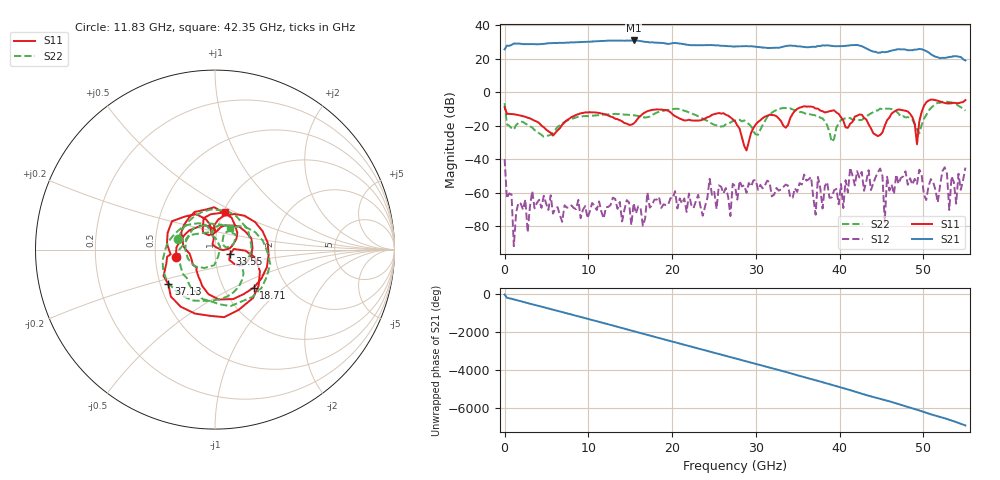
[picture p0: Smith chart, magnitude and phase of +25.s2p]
!Agilent Technologies,E8361C,US49010292,A.09.42.06
!Agilent E8361C: A.09.42.06
!Date: Thursday, December 21, 2023 21:15:18
!Correction: S11(Full 2 Port(1,2))
!S21(Full 2 Port(1,2))
!S12(Full 2 Port(1,2))
!S22(Full 2 Port(1,2))
!S2P File: Measurements: S11, S21, S12, S22:
# Hz S  dB  R 50
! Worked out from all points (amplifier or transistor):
!   201 points, 10 MHz to 55 GHz, reference 50 ohm
!   highest |S21| = 30.9 dB at 15.41 GHz (marker M1)
!   |S21| within 3 dB of that: 674.4 MHz to 25.59 GHz (24.92 GHz wide, 190 % of centre)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
!   unconditionally stable (mu >= 1): start of sweep to end of sweep
!   at 9.083 GHz: K = 84.46, MAG = 30.4 dB, |S12| = -75.3 dB
!   at 27.5 GHz: K = 13.18, MAG = 27.4 dB, |S12| = -56.0 dB
!   at 55 GHz: K = 6.36, MAG = 21.0 dB, |S12| = -45.1 dB
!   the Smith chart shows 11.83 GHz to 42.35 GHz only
!   S11 on the Smith chart (normalised r, x): 11.83 GHz: 0.64, -0.06; 18.71 GHz: 1.38, -0.64; 33.55 GHz: 1.18, -0.06; 37.13 GHz: 0.55, -0.24; 42.35 GHz: 1.02, +0.44
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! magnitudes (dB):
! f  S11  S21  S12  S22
! 10 MHz  -9.0  25.6  -40.0  -6.6
! 1.11 GHz  -13.2  29.1  -92.0  -22.3
! 9.358 GHz  -12.4  30.0  -70.2  -14.3
! 11.83 GHz  -13.1  30.6  -75.5  -13.4
! 15.41 GHz  -18.8  30.9  -66.2  -13.8
! 18.43 GHz  -10.3  29.6  -62.6  -11.7
! 18.71 GHz  -10.4  29.4  -69.2  -11.3
! 27.5 GHz  -17.4  27.3  -56.0  -16.9
! 33.55 GHz  -21.2  27.6  -55.2  -9.5
! 36.85 GHz  -8.9  27.2  -63.0  -13.6
! 37.13 GHz  -9.8  27.1  -73.2  -13.9
! 37.4 GHz  -9.8  27.6  -50.6  -14.0
! 37.95 GHz  -11.4  27.9  -69.5  -15.7
! 42.35 GHz  -13.4  27.9  -51.0  -16.6
! 44.83 GHz  -25.6  23.6  -45.6  -9.8
! 45.38 GHz  -20.1  23.9  -77.5  -9.6
! 45.93 GHz  -15.2  24.5  -58.8  -9.9
! 49.23 GHz  -31.2  25.5  -54.8  -21.8
! 51.7 GHz  -5.1  20.8  -65.9  -6.4
! 52.53 GHz  -6.4  20.5  -44.8  -5.6
! 53.08 GHz  -6.7  21.1  -70.4  -5.9
! 55 GHz  -4.7  18.9  -45.1  -11.0
